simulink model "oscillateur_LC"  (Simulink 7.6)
settings: Solver=ode15s  StartTime=0.0  StopTime=100  RelTol=1e-3
InitFcn:
  | clear all, clc
StopFcn:
  | close all, clc
  | load oscillateur_LC.mat
  | plot(x(1,:),x(2,:))
  | title('Signal de sortie de l''oscillateur RLC et résistance négative')
  | axis([0 100 -1.5e-8 1.5e-8])
  | xlabel('temps')
  | grid
libraries: fl_lib x13, nesl_utility x4, elec_lib x1

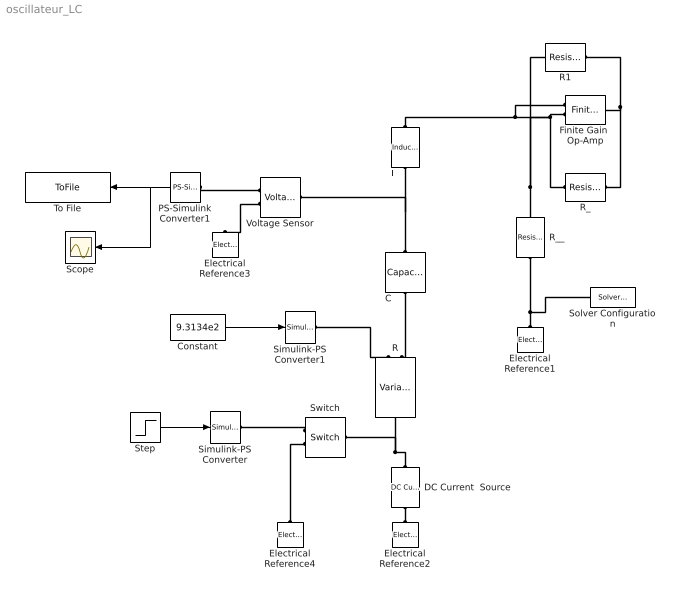
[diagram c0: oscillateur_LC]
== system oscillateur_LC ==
  C : fl_lib/Electrical/Electrical Elements/Capacitor  DialogController=NetworkEngine.DynNeDlgSource  SystemSampleTime=-1  c=10e-3 F  v0=0 V  r=1e-22 Ohm  g=0 1/Ohm  i_Log=off  v_Log=off  vc_Log=off  LocalVarNames=|i|v|vc  LocalVarDescs=|i|v|Internal variable for voltage across capacitor term  LocalVarLogging=[0 0 0]
  Constant : Constant  Value=9.3134e2
  DC Current  Source : fl_lib/Electrical/Electrical Sources/DC Current Source  DialogController=NetworkEngine.DynNeDlgSource  SystemSampleTime=-1  i0=1e-9 A  i_Log=off  v_Log=off  LocalVarNames=|i|v  LocalVarDescs=|i|v  LocalVarLogging=[0 0]
  Electrical Reference{1..4} (4 alike) : fl_lib/Electrical/Electrical Elements/Electrical Reference  DialogController=NetworkEngine.DynNeDlgSource  SystemSampleTime=-1  i_Log=off  LocalVarNames=|i  LocalVarDescs=|i  LocalVarLogging=[]
  Finite Gain  Op-Amp : elec_lib/Integrated Circuits/Finite Gain Op-Amp  DialogController=NetworkEngine.DynNeDlgSource  SystemSampleTime=-1  A=1000  Rin=1e+6 Ohm  Rout=100 Ohm  Vmin=-15 V  Vmax=15 V  LocalVarLogging=[]
  L : fl_lib/Electrical/Electrical Elements/Inductor  DialogController=NetworkEngine.DynNeDlgSource  SystemSampleTime=-1  l=1e-6 H  i0=0 A  r=0 Ohm  g=1e-22 1/Ohm  i_Log=off  v_Log=off  i_L_Log=off  LocalVarNames=|i|v|i_L  LocalVarDescs=|i|v|Internal variable for current through inductor term  LocalVarLogging=[0 0 0]
  PS-Simulink Converter1 : nesl_utility/PS-Simulink Converter  DialogController=NetworkEngine.DynNeUtilDlgSource  SystemSampleTime=-1  PhysicalDomain=network_engine_domain  LeftPortType=input  RightPortType=output  SubClassName=ps_output  Unit=1  AffineConversion=off
  R : fl_lib/Electrical/Electrical Elements/Variable Resistor  DialogController=NetworkEngine.DynNeDlgSource  SystemSampleTime=-1  Rmin=0 Ohm  i_Log=off  v_Log=off  LocalVarNames=|i|v  LocalVarDescs=|i|v  LocalVarLogging=[0 0]
  R1 : fl_lib/Electrical/Electrical Elements/Resistor  DialogController=NetworkEngine.DynNeDlgSource  SystemSampleTime=-1  R=1e3 Ohm  i_Log=off  v_Log=off  LocalVarNames=|i|v  LocalVarDescs=|i|v  LocalVarLogging=[0 0]
  R_ : fl_lib/Electrical/Electrical Elements/Resistor  DialogController=NetworkEngine.DynNeDlgSource  SystemSampleTime=-1  R=10 kOhm  i_Log=off  v_Log=off  LocalVarNames=|i|v  LocalVarDescs=|i|v  LocalVarLogging=[0 0]
  R__ : fl_lib/Electrical/Electrical Elements/Resistor  DialogController=NetworkEngine.DynNeDlgSource  SystemSampleTime=-1  R=10 kOhm  i_Log=off  v_Log=off  LocalVarNames=|i|v  LocalVarDescs=|i|v  LocalVarLogging=[0 0]
  Scope : Scope
  Simulink-PS Converter : nesl_utility/Simulink-PS Converter  DialogController=NetworkEngine.DynNeUtilDlgSource  SystemSampleTime=-1  PhysicalDomain=network_engine_domain  LeftPortType=input  RightPortType=output  SubClassName=ps_input  Unit=1  AffineConversion=off  InputFilterTimeConstant=.001  UdotUserProvided=0
  Simulink-PS Converter1 : nesl_utility/Simulink-PS Converter  DialogController=NetworkEngine.DynNeUtilDlgSource  SystemSampleTime=-1  PhysicalDomain=network_engine_domain  LeftPortType=input  RightPortType=output  SubClassName=ps_input  Unit=1  AffineConversion=off  InputFilterTimeConstant=.001  UdotUserProvided=0
  Solver Configuration : nesl_utility/Solver Configuration  DialogController=NetworkEngine.DynNeUtilDlgSource  SystemSampleTime=-1  PhysicalDomain=network_engine_domain  LeftPortType=input  RightPortType=generic  SubClassName=solver  Accelerate=off  Profile=off  ResidualTolerance=1e-9  MaxNonlinIter=12  MaxModeIter=2  DoFixedCost=off  UseLocalSampling=off  DoDC=off  LinearAlgebra=Sparse  LocalSolverSampleTime=.001  LocalSolverChoice=NE_BACKWARD_EULER_ADVANCER  UseLocalSolver=off
  Step : Step  Time=0.01  SampleTime=0
  Switch : fl_lib/Electrical/Electrical Elements/Switch  DialogController=NetworkEngine.DynNeDlgSource  SystemSampleTime=-1  R_closed=0.01 Ohm  G_open=1e-08 1/Ohm  Threshold=0  i_Log=off  v_Log=off  LocalVarNames=|i|v  LocalVarDescs=|i|v  LocalVarLogging=[0 0]
  To File : ToFile  Filename=oscillateur_LC  MatrixName=x
  Voltage Sensor : fl_lib/Electrical/Electrical Sensors/Voltage Sensor  DialogController=NetworkEngine.DynNeDlgSource  SystemSampleTime=-1  i1_Log=off  v1_Log=off  LocalVarNames=|i1|v1  LocalVarDescs=|i1|v1  LocalVarLogging=[0 0]
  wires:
  PS-Simulink Converter1/1 -> To File/1, Scope/1
  Step/1 -> Simulink-PS Converter/1
  Constant/1 -> Simulink-PS Converter1/1
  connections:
  R_/RConn1 -- R1/RConn1 -- Finite Gain  Op-Amp/RConn1
  Finite Gain  Op-Amp/LConn2 -- R__/LConn1 -- R_/LConn1
  Voltage Sensor/RConn2 -- Electrical Reference3/LConn1
  PS-Simulink Converter1/LConn1 -- Voltage Sensor/RConn1
  L/LConn1 -- R1/LConn1 -- Finite Gain  Op-Amp/LConn1
  Switch/RConn1 -- Simulink-PS Converter/RConn1
  Electrical Reference4/LConn1 -- Switch/RConn2
  DC Current  Source/RConn1 -- Electrical Reference2/LConn1
  DC Current  Source/LConn1 -- Switch/LConn1 -- R/RConn1
  C/RConn1 -- R/LConn2
  C/LConn1 -- L/RConn1 -- Voltage Sensor/LConn1
  Simulink-PS Converter1/RConn1 -- R/LConn1
  Electrical Reference1/LConn1 -- R__/RConn1 -- Solver Configuration/RConn1
